(* Logix 5000 AddOnInstructionDefinition export D_SHR; software revision 30.00 *)

ADD_ON_INSTRUCTION D_SHR   (* revision 1.0 20170524, vendor Kenneth A. Fischer *)
// DINT bit shift right of the 32-bit argument Inp_A by Inp_B bits with paddding by zeros on the right
// Revision note:
// Rev1.0: 20170524 - Initial Release
VAR_IN_OUT
   Inp_A : DINT; {required}   // 64-bit Integer to be right circular rotated
END_VAR
VAR_INPUT
   Inp_B : INT; {required}   // Number of bits to shift
END_VAR
VAR_IN_OUT
   Out : DINT; {required}   // Result
END_VAR
VAR
   BSR_Cntrl : CONTROL := (LEN := 32);
   ONS : BOOL;
   Source_Bit : BOOL;
   Wrk_InpA : DINT[2];
END_VAR

ROUTINE Logic   (* ladder *)
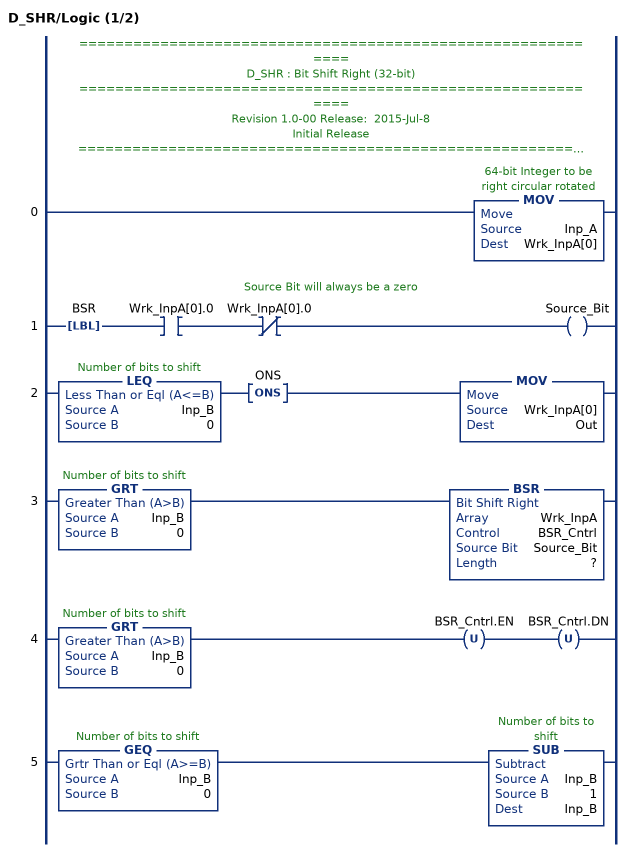
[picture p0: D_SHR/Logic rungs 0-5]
   // ============================================================
   // D_SHR : Bit Shift Right (32-bit)
   // ============================================================
   // Revision 1.0-00 Release:  2015-Jul-8
   // Initial Release
   // ============================================================
   // Performs a right bit shift of the 32-bit argument Inp_A by the
   // number of bits defined in the 16-bit argument Inp_B, with padding by zeros.
   0: MOV(Inp_A,Wrk_InpA[0]);
   // Source Bit will always be a zero
   1: LBL(BSR)XIC(Wrk_InpA[0].0)XIO(Wrk_InpA[0].0)OTE(Source_Bit);
   2: LEQ(Inp_B,0)ONS(ONS)MOV(Wrk_InpA[0],Out);
   3: GRT(Inp_B,0)BSR(Wrk_InpA,BSR_Cntrl,Source_Bit,?);
   4: GRT(Inp_B,0)OTU(BSR_Cntrl.EN)OTU(BSR_Cntrl.DN);
   5: GEQ(Inp_B,0)SUB(Inp_B,1,Inp_B);
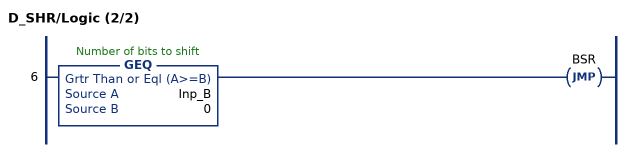
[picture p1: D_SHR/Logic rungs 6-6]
   6: GEQ(Inp_B,0)JMP(BSR);
END_ROUTINE
END_ADD_ON_INSTRUCTION
